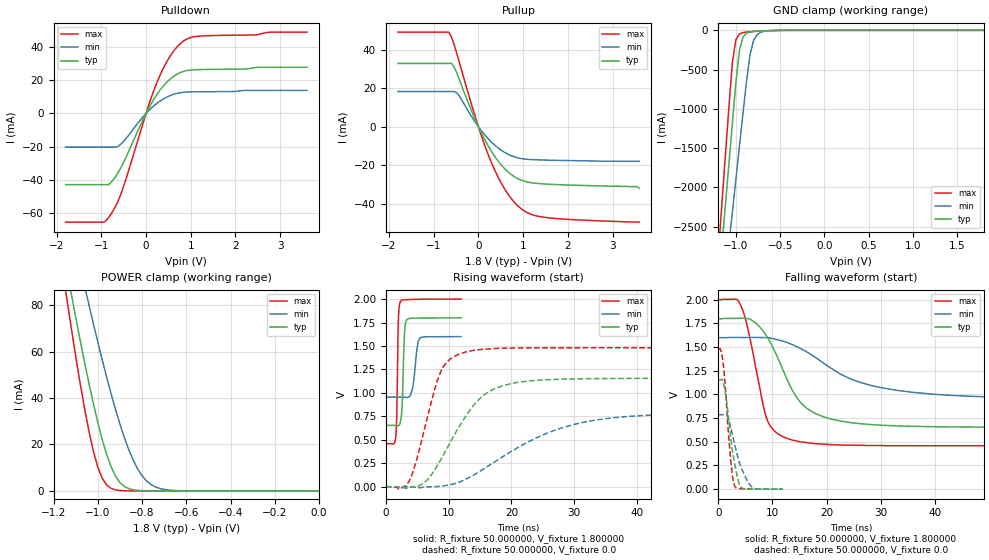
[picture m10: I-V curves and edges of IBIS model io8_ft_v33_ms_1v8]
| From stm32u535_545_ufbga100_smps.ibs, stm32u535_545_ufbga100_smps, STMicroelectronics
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|   Model io8_ft_v33_ms_1v8
[Model]  io8_ft_v33_ms_1v8
Model_type I/O
Polarity   Non-Inverting
Enable   Active-Low
Vinl =   0.540000V
Vinh =   1.260000V
Vmeas =  0.900000V
Cref =   50.000000pF
Rref =   100.000000M
Vref =   0.0V
C_comp   3.087500pF   3.086600pF   3.135700pF
[Temperature Range]   25.000000   0.140000k   -40.000000
[Pullup Reference]   1.800000V   1.600000V   2.000000V
[Pulldown Reference]   0.0V   0.0V   0.0V
[POWER Clamp Reference]   1.800000V   1.600000V   2.000000V
[GND Clamp Reference]   0.0V   0.0V   0.0V
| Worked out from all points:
|   slope of the pulldown table from 0 to 0.27 V, typ, clamps not added: 21.7 ohm
|   slope of the pullup table from 0 to 0.27 V, typ, clamps not added: 22.6 ohm
|   GND clamp passes 1 mA (typ) near -0.51 V on its own axis
|   POWER clamp passes 1 mA (typ) near -0.86 V on its own axis
|   rising waveform, R_fixture 50.000000, V_fixture 1.800000: 20-80 % time 316ps typ, 628ps min, 226ps max; typ from 0.654 V to 1.8 V
|   rising waveform, R_fixture 50.000000, V_fixture 0.0: 20-80 % time 6.48ns typ, 13.4ns min, 3.57ns max; typ from 0 V to 1.16 V
|   falling waveform, R_fixture 50.000000, V_fixture 1.800000: 20-80 % time 6.36ns typ, 13.4ns min, 3.35ns max; typ from 1.8 V to 0.654 V
|   falling waveform, R_fixture 50.000000, V_fixture 0.0: 20-80 % time 1.6ns typ, 2.38ns min, 1.18ns max; typ from 1.16 V to 0 V
[Pulldown]
|Voltage   I(typ)   I(min)   I(max)
-1.8V     -42.74mA   -20.21mA   -65.25mA
-960mV    -42.74mA   -20.21mA   -65.25mA
-780mV    -41.3mA    -20.21mA   -60.25mA
-660mV    -37mA      -20.2mA    -54.5mA
-540mV    -31.39mA   -17.82mA   -46.65mA
0V        -10fA      0A         10fA
240mV     11.28mA    6.002mA    18.38mA
480mV     19.18mA    10.02mA    31.83mA
780mV     24.67mA    12.5mA     42.21mA
960mV     25.9mA     12.9mA     45.21mA
1.14V     26.24mA    12.99mA    46.23mA
3.6V      27.69mA    13.82mA    48.79mA
[Pullup]
|Voltage   I(typ)   I(min)   I(max)
-1.8V     32.87mA    18.3mA     49.14mA
-660mV    32.87mA    18.3mA     49.14mA
-600mV    32.87mA    18.3mA     46.41mA
-480mV    27.73mA    17.56mA    37.8mA
-60mV     3.108mA    1.975mA    4.436mA
240mV     -10.82mA   -6.752mA   -15.73mA
420mV     -17.18mA   -10.64mA   -25.23mA
600mV     -22.1mA    -13.54mA   -32.82mA
960mV     -27.82mA   -16.55mA   -42.66mA
1.2V      -29.16mA   -17.09mA   -45.68mA
1.56V     -29.85mA   -17.38mA   -47.3mA
3.6V      -32mA      -18mA      -49.6mA
[GND_clamp]
|Voltage   I(typ)   I(min)   I(max)
-1.8V     -9.707A    -9.942A    -9.774A
-1.2V     -3.309A    -4.006A    -2.864A
-1.16V    -2.777A    -3.584A    -2.239A
-1.12V    -2.246A    -3.162A    -1.614A
-1.04V    -1.186A    -2.319A    -408.6mA
-1V       -663.9mA   -1.898A    -117.8mA
-960mV    -254mA     -1.478A    -45.14mA
-920mV    -86.03mA   -1.06A     -28.58mA
-840mV    -19.12mA   -308.9mA   -18.74mA
-800mV    -13.39mA   -130.8mA   -15.31mA
-720mV    -7.948mA   -25.37mA   -9.381mA
1.8V      0A         14.97nA    0A
[POWER_clamp]
|Voltage   I(typ)   I(min)   I(max)
-1.8V     470.8mA    433.7mA    554.6mA
-1.14V    95.25mA    122.7mA    82.82mA
-1.12V    84.97mA    114mA      70.27mA
-1.06V    55.51mA    88.42mA    35.67mA
-1.04V    46.34mA    80.15mA    25.76mA
-1V       29.51mA    64.13mA    10.3mA
-940mV    10.39mA    41.86mA    1.109mA
-900mV    3.624mA    28.77mA    182.8uA
-840mV    490.7uA    13.24mA    11.35uA
-800mV    116.8uA    6.532mA    1.77uA
-740mV    13.2uA     1.723mA    109.3nA
0V        0A         18.72nA    0A
[Ramp]
| variable   typ   min   max
dV/dt_r  0.69300/6.47285n   0.47200/13.35286n   0.88872/3.56422n
dV/dt_f  0.68765/6.34922n   0.38599/13.40723n   0.92481/3.34940n
R_load = 50.000000
[Rising Waveform]
R_fixture= 50.000000
V_fixture= 1.800000
V_fixture_min= 1.600000
V_fixture_max= 2.000000
|time   V(typ)   V(min)   V(max)
0s        654mV      955.4mV    458.7mV
1.586ns   653.4mV    955.4mV    541.7mV
1.73ns    652.2mV    955.4mV    759.6mV
1.994ns   651mV      955.4mV    1.776V
2.33ns    698.2mV    955.4mV    1.975V
2.619ns   901.1mV    955.2mV    1.989V
2.979ns   1.646V     954.1mV    1.993V
3.315ns   1.777V     951.7mV    1.994V
5.405ns   1.798V     1.582V     1.998V
11.96ns   1.8V       1.6V       2V
[Rising Waveform]
R_fixture= 50.000000
V_fixture= 0.0
V_fixture_min= 0.0
V_fixture_max= 0.0
|time   V(typ)   V(min)   V(max)
0s        4.581uV    -1.107uV   13.17uV
3.524ns   -10.55mV   -392uV     40.55mV
6.246ns   51.54mV    -2.601mV   641.8mV
8.809ns   296.9mV    6.05mV     1.238V
12.81ns   761.3mV    83.21mV    1.438V
15.86ns   990mV      201.9mV    1.467V
18.74ns   1.08V      326mV      1.476V
26.75ns   1.143V     598.5mV    1.481V
33.79ns   1.153V     714.5mV    1.481V
79.76ns   1.155V     786.8mV    1.481V
[Falling Waveform]
R_fixture= 50.000000
V_fixture= 1.800000
V_fixture_min= 1.600000
V_fixture_max= 2.000000
|time   V(typ)   V(min)   V(max)
0s        1.8V       1.6V       2V
4.004ns   1.805V     1.603V     1.959V
5.445ns   1.801V     1.603V     1.703V
8.969ns   1.613V     1.6V       745.3mV
13.45ns   1.069V     1.531V     522mV
15.86ns   878.3mV    1.465V     495mV
18.9ns    775.7mV    1.353V     476.9mV
24.5ns    702.5mV    1.163V     464.4mV
33.15ns   668.1mV    1.043V     459.6mV
79.76ns   654mV      955.4mV    458.7mV
[Falling Waveform]
R_fixture= 50.000000
V_fixture= 0.0
V_fixture_min= 0.0
V_fixture_max= 0.0
|time   V(typ)   V(min)   V(max)
0s        1.155V     786.8mV    1.481V
432.4ps   1.155V     786.8mV    1.474V
961ps     1.123V     786.6mV    1.306V
1.586ns   917.3mV    786.8mV    845.2mV
2.282ns   558.3mV    661mV      328.8mV
2.715ns   371.9mV    555.4mV    109.4mV
3.051ns   266.8mV    471.7mV    30.26mV
4.06ns    32.15mV    254.4mV    4.584mV
6.318ns   1.79mV     17.84mV    807.4uV
11.96ns   4.581uV    -1.107uV   13.17uV
